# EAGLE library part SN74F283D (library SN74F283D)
4-BITBIN FULL ADDER Source: Datasheet
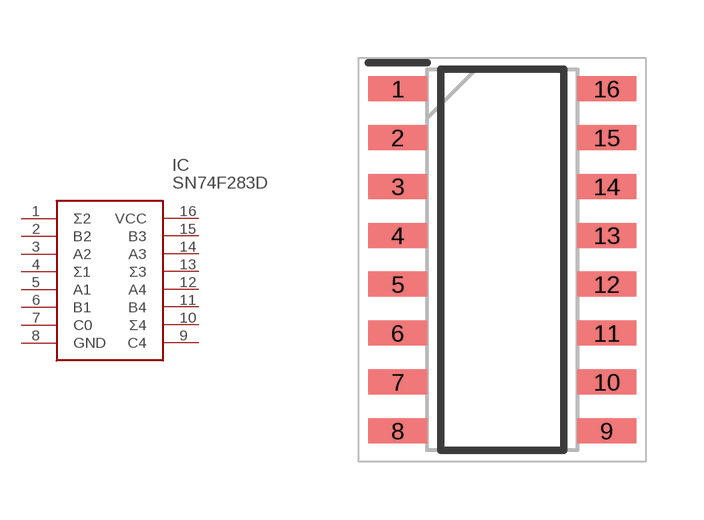
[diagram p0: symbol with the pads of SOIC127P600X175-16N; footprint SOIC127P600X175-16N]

Designator prefix IC

## SN74F283D (Description: 4-BITBIN FULL ADDER; Height: 1.75mm; Manufacturer_Name: Texas Instruments; Manufacturer_Part_Number: SN74F283D; Mouser_Part_Number: 595-SN74F283D; Mouser_Price-Stock: https://www.mouser.co.uk/ProductDetail/Texas-Instruments/SN74F283D?qs=RnzODY3cU8t9RP7%252BwWjEZw%3D%3D)  [SOIC127P600X175-16N]
1  Σ2
2  B2
3  A2
4  Σ1
5  A1
6  B1
7  C0
8  GND
9  C4
10  Σ4
11  B4
12  A4
13  Σ3
14  A3
15  B3
16  VCC

## Footprint SOIC127P600X175-16N (pad centres in mm)
D (R-PDSO-G16)
smd 1.525 x 0.65: 1 -2.712,4.445; 2 -2.712,3.175; 3 -2.712,1.905; 4 -2.712,0.635; 5 -2.712,-0.635; 6 -2.712,-1.905; 7 -2.712,-3.175; 8 -2.712,-4.445; 9 2.712,-4.445; 10 2.712,-3.175; 11 2.712,-1.905; 12 2.712,-0.635; 13 2.712,0.635; 14 2.712,1.905; 15 2.712,3.175; 16 2.712,4.445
